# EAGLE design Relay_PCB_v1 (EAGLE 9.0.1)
Relay1
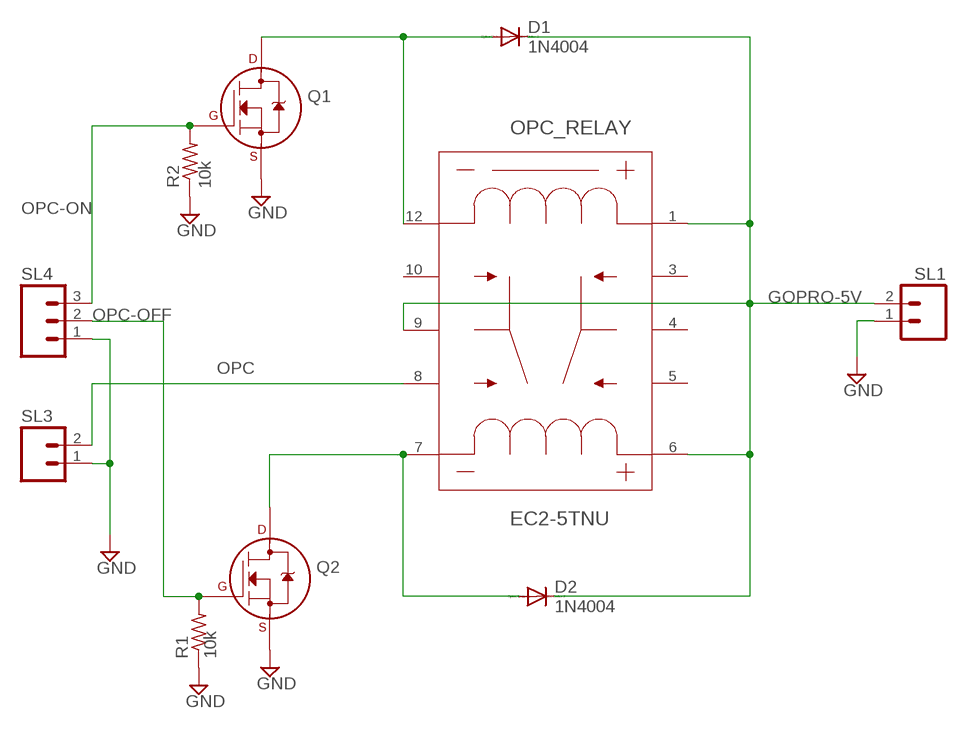
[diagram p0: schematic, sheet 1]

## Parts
D1  1N4004  [DO41-10]
D2  1N4004  [DO41-10]
OPC_RELAY  EC2-5TNU  [EC2TNU]
Q1  2N7000_TO92  [TO-92]
Q2  2N7000_TO92  [TO-92]
R1  R-US_0207/7  [0207/7]
R2  R-US_0207/7  [0207/7]
SL1  M02  [02P]
SL3  M02  [02P]
SL4  M03  [03P]

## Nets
GND: Q1.1(S) Q2.1(S) R1.1 R2.1 SL1.1 SL3.1 SL4.1
GOPRO-5V: D1.C D2.C OPC_RELAY.1 OPC_RELAY.6 OPC_RELAY.9 SL1.2
N$1: D1.A OPC_RELAY.12 Q1.3(D)
N$3: D2.A OPC_RELAY.7 Q2.3(D)
OPC: OPC_RELAY.8 SL3.2
OPC-OFF: Q2.2(G) R1.2 SL4.2
OPC-ON: Q1.2(G) R2.2 SL4.3
Unconnected: OPC_RELAY.3 OPC_RELAY.4 OPC_RELAY.5 OPC_RELAY.10

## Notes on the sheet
- 10k
- 10k

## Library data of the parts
D1 D2 = diode:1N4004: DIODE
OPC_RELAY = EC2-5TNU:EC2-5TNU; MANUFACTURER_PART_NUMBER: EC25TNU; VENDOR: KEMET
Q1 Q2 = transistors:2N700*: 2N7000, 2N7002, NDS7002A N-channel enhancement mode MOSFET
R1 R2 = rcl:R-US_: RESISTOR, American symbol; SPICEPREFIX: R
SL1 SL3 = con-amp-quick:M02: AMP QUICK CONNECTOR; OC_FARNELL: unknown; OC_NEWARK: unknown
SL4 = con-amp-quick:M03: AMP QUICK CONNECTOR; OC_FARNELL: unknown; OC_NEWARK: unknown

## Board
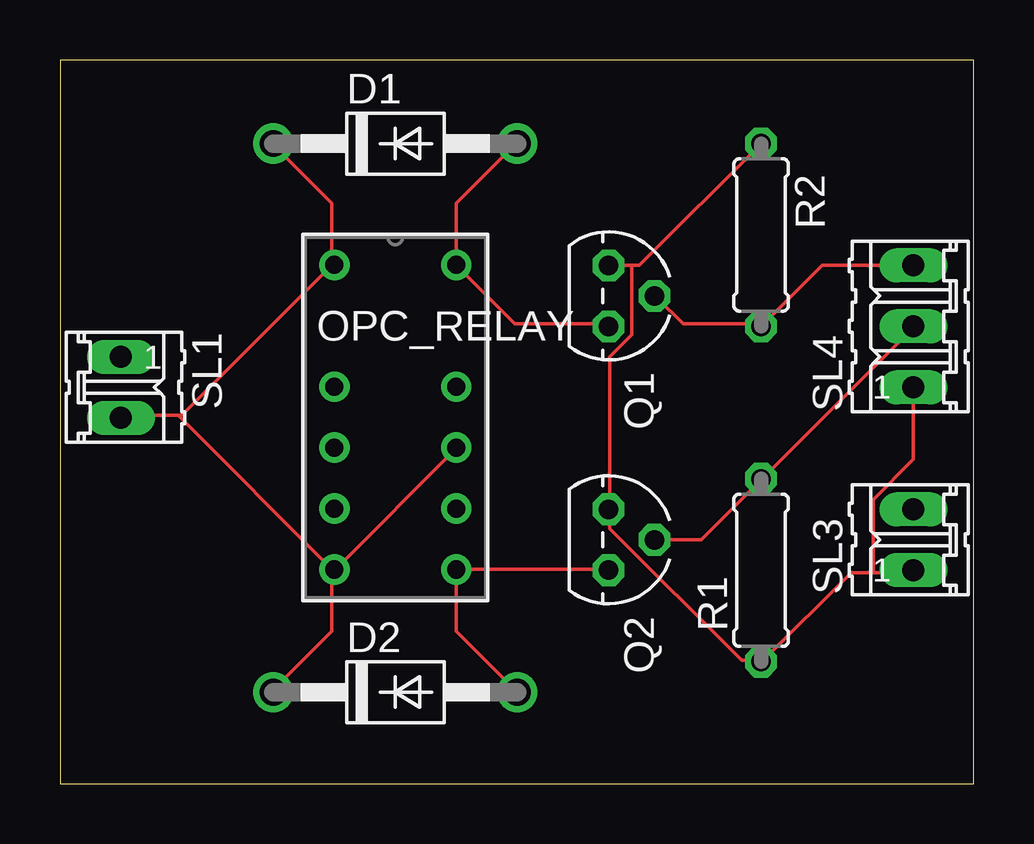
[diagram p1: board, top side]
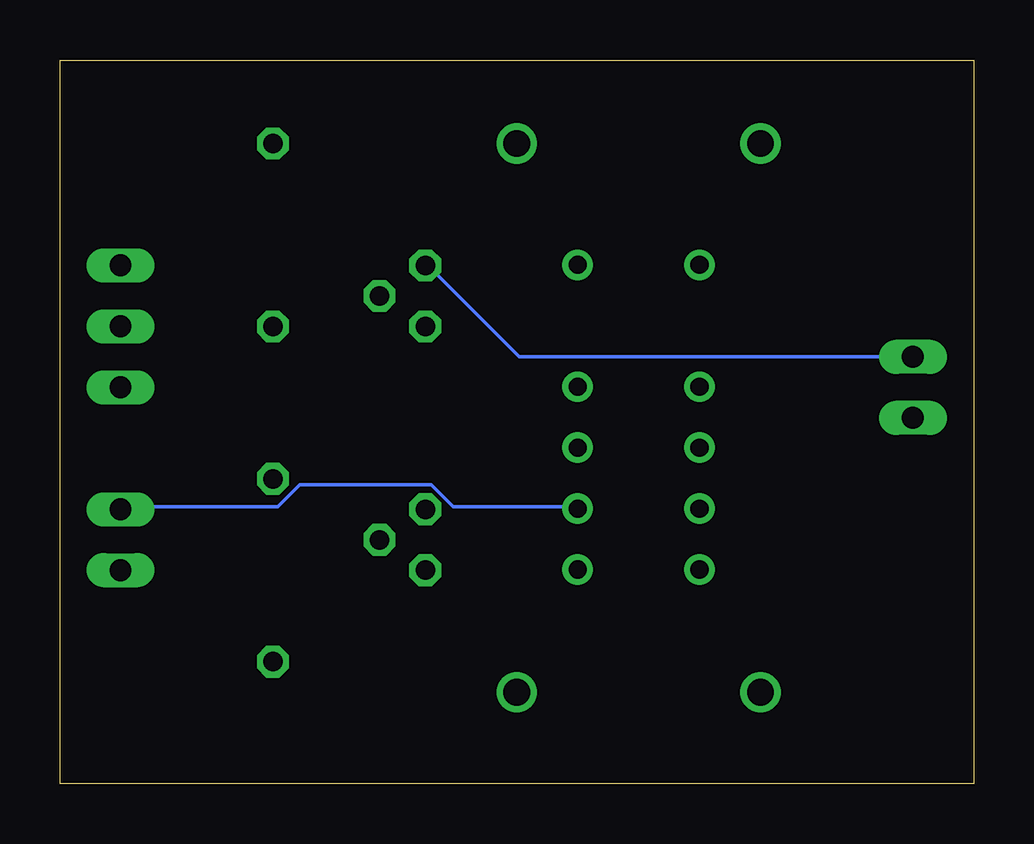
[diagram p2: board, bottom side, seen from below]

Size 38.08 x 30.15 mm. Coordinates in mm from the lower left corner, seen from the top.
Outline: 0,0 38.08,0 38.08,30.15 0,30.15 0,0
Copper layers (1*16): Top 0.035mm / dielectric 1.5mm / Bottom 0.035mm
Design rules "default": minimum track width 6mil, minimum drill 0.35mm, track to track 6mil, track to pad 6mil, pad to pad 6mil, via to via 6mil, smd to smd 6mil, copper to edge 40mil, drill to drill 6mil, minimum pad ring 10mil, minimum via ring 8mil, stop-mask expansion 4mil, vias tented up to drill 0mil, thermal gap 10mil

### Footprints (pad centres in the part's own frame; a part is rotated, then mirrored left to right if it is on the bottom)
DO41-10 = drill 1.118: A 5.08,0; C -5.08,0
EC2TNU = drill 0.762 pad 1.27: 1 -2.54,6.375; 3 -2.54,1.295; 4 -2.54,-1.245; 5 -2.54,-3.785; 6 -2.54,-6.325; 7 2.54,-6.325; 8 2.54,-3.785; 9 2.54,-1.245; 10 2.54,1.295; 12 2.54,6.375
TO-92 = drill 0.813 octagon: 1 -1.27,0; 2 0,1.905; 3 1.27,0
0207/7 = drill 0.813 octagon: 1 -3.81,0; 2 3.81,0
02P = drill 0.914 long: 1 -1.27,0; 2 1.27,0
03P = drill 0.914 long: 1 -2.54,0; 2 0,0; 3 2.54,0

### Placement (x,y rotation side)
D1  13.97,26.67 0 top
D2  13.97,3.81 0 top
OPC_RELAY  13.97,15.24 0 top
Q1  22.86,20.32 270 top
Q2  22.86,10.16 270 top
R1  29.21,8.89 90 top
R2  29.21,22.86 270 top
SL1  2.54,16.51 270 top
SL3  35.56,10.16 90 top
SL4  35.56,19.05 90 top

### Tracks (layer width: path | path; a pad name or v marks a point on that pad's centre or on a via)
GND
  Top 0.152: 33.88,8.79 32.97,8.79 29.31,5.13 R1.1 29.16,5.13 28.4,5.13 22.91,10.62 22.91,11.38 Q2.1 22.91,11.53 22.91,17.78 23.82,18.69 23.82,21.59 | 33.88,8.79 35.56,8.79 SL3.1 | SL4.1 35.56,13.51 33.88,11.84 33.88,8.79 | 23.82,21.59 24.13,21.59 R2.1 | 23.82,21.59 Q1.1
  Bottom 0.152: SL1.1 18.95,17.78 22.76,21.59 Q1.1
GOPRO-5V
  Top 0.152: OPC_RELAY.6 11.33,8.79 11.33,6.35 8.89,3.91 D2.C | OPC_RELAY.9 16.51,13.97 11.48,8.94 OPC_RELAY.6 | D1.C 8.89,26.62 11.33,24.18 11.33,21.74 OPC_RELAY.1 11.33,21.59 5.08,15.34 4.93,15.34 | 4.93,15.34 2.64,15.34 SL1.2 | 4.93,15.34 11.33,8.94 OPC_RELAY.6
N$1
  Top 0.152: D1.A 18.95,26.62 16.51,24.18 OPC_RELAY.12 16.51,21.59 18.95,19.15 22.76,19.15 Q1.3
N$3
  Top 0.152: D2.A 16.51,6.35 OPC_RELAY.7 16.51,8.94 22.76,8.94 Q2.3
OPC
  Bottom 0.152: OPC_RELAY.8 16.51,11.53 21.69,11.53 22.61,12.45 28.09,12.45 29.01,11.53 35.56,11.53 SL3.2
OPC-OFF
  Top 0.152: Q2.2 26.72,10.16 29.16,12.6 R1.2 29.31,12.75 35.56,19 SL4.2
OPC-ON
  Top 0.152: Q1.2 24.89,20.22 25.96,19.15 29.16,19.15 R2.2 31.75,21.59 SL4.3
